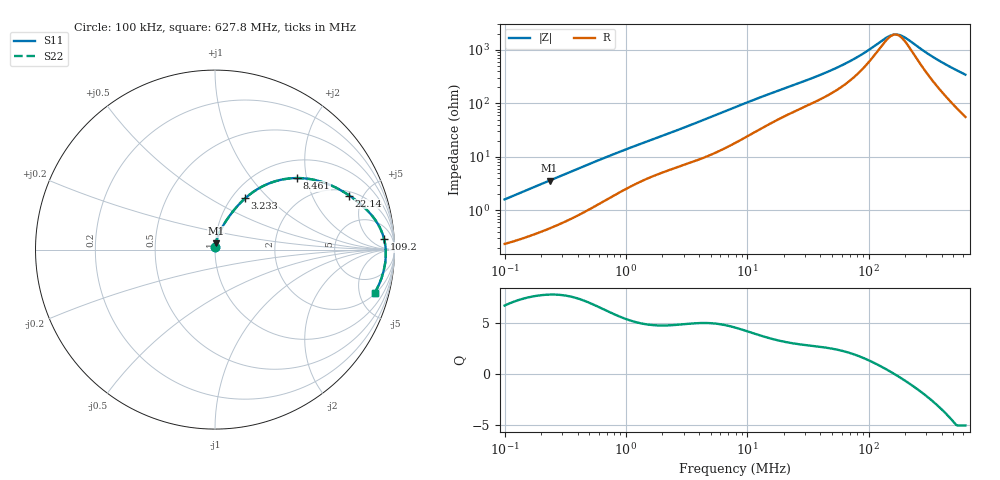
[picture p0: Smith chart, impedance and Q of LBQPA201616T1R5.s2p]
! LBQPA201616T1R5  S-PARAMETER MODEL  ( General Type )
! Model Generated by TAIYO YUDEN Corporation (http://www.ty-top.com)
! Version 1.0
! TAIYO YUDEN Control No. 191025NI43SB-FBB
! Copyright(c) 2019 TAIYO YUDEN CO.,LTD. All Rights Reserved.
! Product Description (link to TY-COMPAS)
! https://ds.yuden.co.jp/TYCOMPAS/or/detail?pn=LBQPA201616T1R5M&u=M
! Products Name : Inductors
! Characteristics :
!  Inductance : 1.5 uH , SRF(min) : 80 MHz , DC Resistance(max) : 0.195 Ohm
!  Rated Current : Saturation :1000 mA , Temp Rise : 775 mA (20 degC)
!  Case Size : 2.0 x 1.6 / 0.079 x 0.063 [mm/inch] , Thickness : 1.6 / 0.063 [mm/inch]
!  (Conditions: Temperature = 25 degC , DC Bias Current/Voltage = 0A / 0V)
! External Node Assignments :
!  1  o---GGG---o  2
! GND o---------o GND
! Frequency Range : 0.1MHz  -  627.813588MHz  [ 402 STEP ]
# MHz S RI R 50
! Freq[MHz].  S11 Real  S11 Imag  S21 Real  S21 Imag  S12 Real  S12 Imag  S22 Real  S22 Imag
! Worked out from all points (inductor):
!   401 points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, 100 kHz to 627.8 MHz, reference 50 ohm
!   read as one part in series: L = 2.5 uH near 104.5 kHz
!   highest Q = 7.78 at 234.6 kHz (marker M1), where L = 2.43 uH
!   self-resonance near 164.5 MHz
!   S11 on the Smith chart (normalised r, x): 100 kHz: 1.00, +0.03; 3.233 MHz: 1.15, +0.74; 8.461 MHz: 1.39, +1.76; 22.14 MHz: 2.27, +3.91; 109.2 MHz: 16, +17; 627.8 MHz: 2.12, -6.80
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0.1  0.00261 0.0158  0.9974 -0.0158  0.9974 -0.0158  0.00261 0.0158
0.234579  0.00585 0.0355  0.9942 -0.0355  0.9942 -0.0355  0.00585 0.0355
0.43265  0.0127 0.0625  0.9873 -0.0625  0.9873 -0.0625  0.0127 0.0625
0.950477  0.0387 0.1222  0.9613 -0.1222  0.9613 -0.1222  0.0387 0.1222
1.87186  0.09 0.1999  0.91 -0.1999  0.91 -0.1999  0.09 0.1999
3.233238  0.1675 0.2854  0.8325 -0.2854  0.8325 -0.2854  0.1675 0.2854
4.898179  0.2682 0.3541  0.7318 -0.3541  0.7318 -0.3541  0.2682 0.3541
7.923469  0.4326 0.3979  0.5674 -0.3979  0.5674 -0.3979  0.4326 0.3979
8.46056  0.457 0.3987  0.543 -0.3987  0.543 -0.3987  0.457 0.3987
13.9886  0.6302 0.3649  0.3698 -0.3649  0.3698 -0.3649  0.6302 0.3649
22.13913  0.7482 0.3013  0.2518 -0.3013  0.2518 -0.3013  0.7482 0.3013
34.28088  0.8304 0.2361  0.1696 -0.2361  0.1696 -0.2361  0.8304 0.2361
47.58506  0.8775 0.1859  0.1225 -0.1859  0.1225 -0.1859  0.8775 0.1859
64.62413  0.91 0.1382  0.09 -0.1382  0.09 -0.1382  0.91 0.1382
84.00974  0.9294 0.098  0.0706 -0.098  0.0706 -0.098  0.9294 0.098
109.2105  0.942 0.059  0.058 -0.059  0.058 -0.059  0.942 0.059
148.3162  0.9498 0.0149  0.0502 -0.0149  0.0502 -0.0149  0.9498 0.0149
169.1049  0.9512 -0.00399  0.0488 0.00399  0.0488 0.00399  0.9512 -0.00399
192.8073  0.9517 -0.0231  0.0483 0.0231  0.0483 0.0231  0.9517 -0.0231
355.6082  0.9386 -0.1224  0.0614 0.1224  0.0614 0.1224  0.9386 -0.1224
482.9429  0.9184 -0.1832  0.0816 0.1832  0.0816 0.1832  0.9184 -0.1832
627.8136  0.8887 -0.243  0.1113 0.243  0.1113 0.243  0.8887 -0.243
